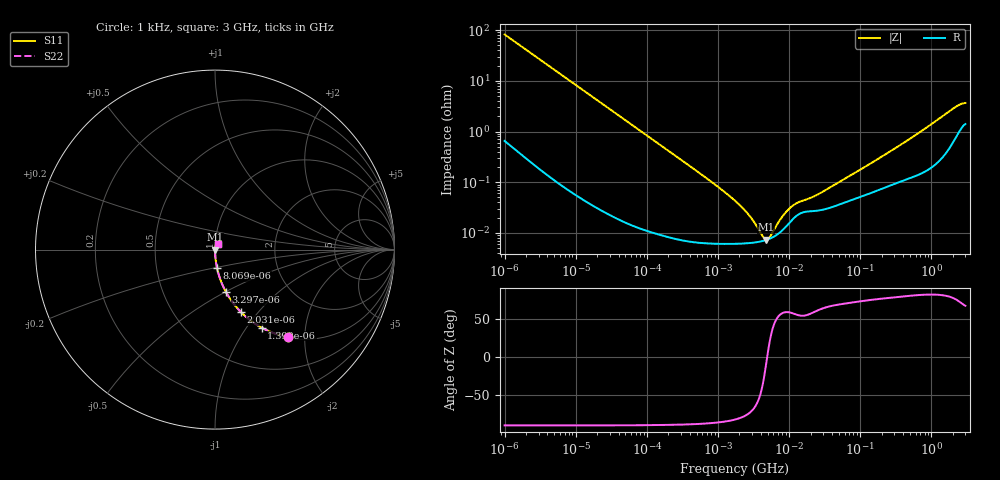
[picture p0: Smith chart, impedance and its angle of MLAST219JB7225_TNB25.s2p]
! MLAST219JB7225_TNB25  S-PARAMETER MODEL  ( Standard Model )
! Model Generated by TAIYO YUDEN Corporation (http://www.ty-top.com)
! Version 1.0
! TAIYO YUDEN Control No. 220601
! Copyright(c) 2011 TAIYO YUDEN CO.,LTD. All Rights Reserved.
! Product Description (link to TY-COMPAS)
! https://ds.yuden.co.jp/TYCOMPAS/or/detail?pn=MLAST219JB7225KTNB25&u=M
! Products Name : Multilayer Ceramic Capacitors
! Characteristics :
!  Capacitance : 2.2 [uF] , Rated Voltage : 25 [V] , TCC : X7R
!  Case Size : 2.0 x 1.25 / 0.079 x 0.049 [mm/inch] , Thickness : 0.85 / 0.033 [mm/inch]
!  (Conditions: Temperature = 25 [degC] , DC Bias Voltage = 0 [V])
! External Node Assignments :
!  1  o---| |---o  2
! GND o---------o GND
! Frequency Range : 1kHz  -  3GHz  [ 401 STEP ]
# MHZ S RI R 50
! Freq[MHz].  S11 Real  S11 Imag  S21 Real  S21 Imag  S12 Real  S12 Imag  S22 Real  S22 Imag
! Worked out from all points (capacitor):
!   401 points, 1 kHz to 3 GHz, reference 50 ohm
!   read as one part in series: C = 1.93 uF near 1.077 kHz
!   lowest |Z| = 7.35 mohm at 4.74 MHz (marker M1)
!   series resonance near 4.906 MHz, so ESL is about 540 pH
!   S11 on the Smith chart (normalised r, x): 1 kHz: 1.01, -1.64; 1.399 kHz: 1.01, -1.18; 2.031 kHz: 1.01, -0.81; 3.297 kHz: 1.00, -0.50; 8.069 kHz: 1.00, -0.21; 3 GHz: 1.03, +0.07
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0.001  0.4042 -0.4868  0.5958 0.4868  0.5958 0.4868  0.4042 -0.4868
0.001399  0.2591 -0.4344  0.7409 0.4344  0.7409 0.4344  0.2591 -0.4344
0.002031  0.1435 -0.347  0.8565 0.347  0.8565 0.347  0.1435 -0.347
0.003297  0.0606 -0.2352  0.9394 0.2352  0.9394 0.2352  0.0606 -0.2352
0.008069  0.0111 -0.1016  0.9889 0.1016  0.9889 0.1016  0.0111 -0.1016
0.01216  0.00511 -0.0679  0.9949 0.0679  0.9949 0.0679  0.00511 -0.0679
0.033275  0.000836 -0.025  0.9992 0.025  0.9992 0.025  0.000836 -0.025
0.147855  0.000125 -0.00567  0.9999 0.00567  0.9999 0.00567  0.000125 -0.00567
0.791611  6.27e-05 -0.00104  0.9999 0.00104  0.9999 0.00104  6.27e-05 -0.00104
1.732051  6.11e-05 -0.000427  0.9999 0.000427  0.9999 0.000427  6.11e-05 -0.000427
2.709407  6.3e-05 -0.000218  0.9999 0.000218  0.9999 0.000218  6.3e-05 -0.000218
3.93371  6.77e-05 -7.75e-05  0.9999 7.75e-05  0.9999 7.75e-05  6.77e-05 -7.75e-05
4.739869  7.25e-05 -1.2e-05  0.9999 1.2e-05  0.9999 1.2e-05  7.25e-05 -1.2e-05
5.502215  7.85e-05 4.03e-05  0.9999 -4.03e-05  0.9999 -4.03e-05  7.85e-05 4.03e-05
5.928204  8.27e-05 6.68e-05  0.9999 -6.68e-05  0.9999 -6.68e-05  8.27e-05 6.68e-05
8.291982  0.000118 0.00019  0.9999 -0.00019  0.9999 -0.00019  0.000118 0.00019
11.1738  0.000185 0.00029  0.9998 -0.00029  0.9998 -0.00029  0.000185 0.00029
13.46371  0.000231 0.000329  0.9998 -0.000329  0.9998 -0.000329  0.000231 0.000329
21.06097  0.000269 0.000429  0.9997 -0.000429  0.9997 -0.000429  0.000269 0.000429
256.0921  0.000862 0.00387  0.9991 -0.00387  0.9991 -0.00387  0.000862 0.00387
2144.796  0.00791 0.0288  0.9921 -0.0288  0.9921 -0.0288  0.00791 0.0288
3000  0.015 0.0327  0.985 -0.0327  0.985 -0.0327  0.015 0.0327
